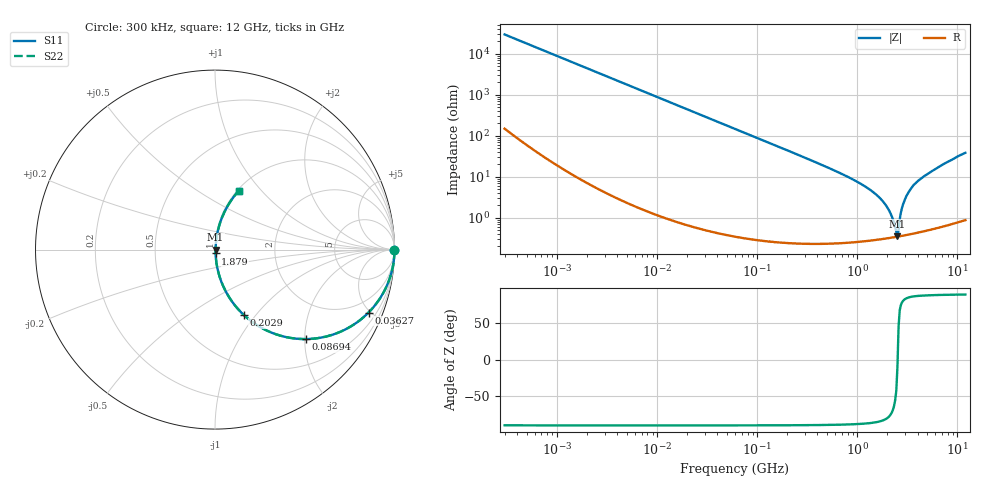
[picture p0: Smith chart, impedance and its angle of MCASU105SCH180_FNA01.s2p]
! MCASU105SCH180_FNA01  S-PARAMETER MODEL  ( General Type )
! Model Generated by TAIYO YUDEN Corporation (http://www.ty-top.com)
! Version 1.0
! TAIYO YUDEN Control No. 130207
! Copyright(c) 2013 TAIYO YUDEN CO.,LTD. All Rights Reserved.
! Product Description (link to TY-COMPAS)
! https://ds.yuden.co.jp/TYCOMPAS/or/detail?pn=MCASU105SCH180JFNA01&u=M
! Products Name : Multilayer Ceramic Capacitors
! Characteristics :
!  Capacitance : 18 pF , Rated Voltage : 50V , TCC : CH / C0H
!  Case Size : 1.0 x 0.5 / 0.039 x 0.02 [mm/inch] , Thickness : 0.5 / 0.02 [mm/inch]
!  (Conditions: Temperature = 25 degC , DC Bias Current/Voltage = 0A / 0V)
! External Node Assignments :
!  1  o---| |---o  2
! GND o---------o GND
! Frequency Range : 300000Hz  -  12GHz  [ 401 STEP ]
# MHz S RI R 50
! Freq[MHz].  S11 Real  S11 Imag  S21 Real  S21 Imag  S12 Real  S12 Imag  S22 Real  S22 Imag
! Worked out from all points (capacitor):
!   401 points, 300 kHz to 12 GHz, reference 50 ohm
!   read as one part in series: C = 18 pF near 316.3 kHz
!   lowest |Z| = 351 mohm at 2.514 GHz (marker M1)
!   series resonance near 2.524 GHz, so ESL is about 220 pH
!   S11 on the Smith chart (normalised r, x): 300 kHz: open; 36.27 MHz: 1.01, -4.88; 86.94 MHz: 1.01, -2.03; 202.9 MHz: 1.00, -0.87; 1.879 GHz: 1.01, -0.04; 12 GHz: 1.02, +0.77
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0.3  1 -0.00339  2.86e-05 0.00339  2.86e-05 0.00339  1 -0.00339
1.769972  0.9996 -0.02  0.000433 0.02  0.000433 0.02  0.9996 -0.02
10.44266  0.9861 -0.1164  0.0139 0.1164  0.0139 0.1164  0.9861 -0.1164
36.27049  0.8555 -0.3507  0.1445 0.3507  0.1445 0.3507  0.8555 -0.3507
60  0.6842 -0.4637  0.3158 0.4637  0.3158 0.4637  0.6842 -0.4637
86.94074  0.508 -0.4985  0.492 0.4985  0.492 0.4985  0.508 -0.4985
202.9496  0.1593 -0.3632  0.8407 0.3632  0.8407 0.3632  0.1593 -0.3632
353.9943  0.0586 -0.2302  0.9414 0.2302  0.9414 0.2302  0.0586 -0.2302
1076.992  0.00711 -0.067  0.9929 0.067  0.9929 0.067  0.00711 -0.067
1480.043  0.0044 -0.0395  0.9956 0.0395  0.9956 0.0395  0.0044 -0.0395
1878.541  0.00354 -0.0216  0.9965 0.0216  0.9965 0.0216  0.00354 -0.0216
2088.533  0.00339 -0.0141  0.9966 0.0141  0.9966 0.0141  0.00339 -0.0141
2384.334  0.00339 -0.00492  0.9966 0.00492  0.9966 0.00492  0.00339 -0.00492
2448.343  0.00341 -0.00316  0.9966 0.00316  0.9966 0.00316  0.00341 -0.00316
2514.07  0.00344 -0.000617  0.9966 0.000617  0.9966 0.000617  0.00344 -0.000617
2581.562  0.00349 0.00348  0.9965 -0.00348  0.9965 -0.00348  0.00349 0.00348
2795.104  0.00389 0.017  0.9961 -0.017  0.9961 -0.017  0.00389 0.017
2947.191  0.00433 0.0253  0.9957 -0.0253  0.9957 -0.0253  0.00433 0.0253
3276.641  0.00571 0.0427  0.9943 -0.0427  0.9943 -0.0427  0.00571 0.0427
3740.715  0.00845 0.0653  0.9916 -0.0653  0.9916 -0.0653  0.00845 0.0653
6354.153  0.0324 0.1611  0.9676 -0.1611  0.9676 -0.1611  0.0324 0.1611
12000  0.1334 0.3288  0.8666 -0.3288  0.8666 -0.3288  0.1334 0.3288
